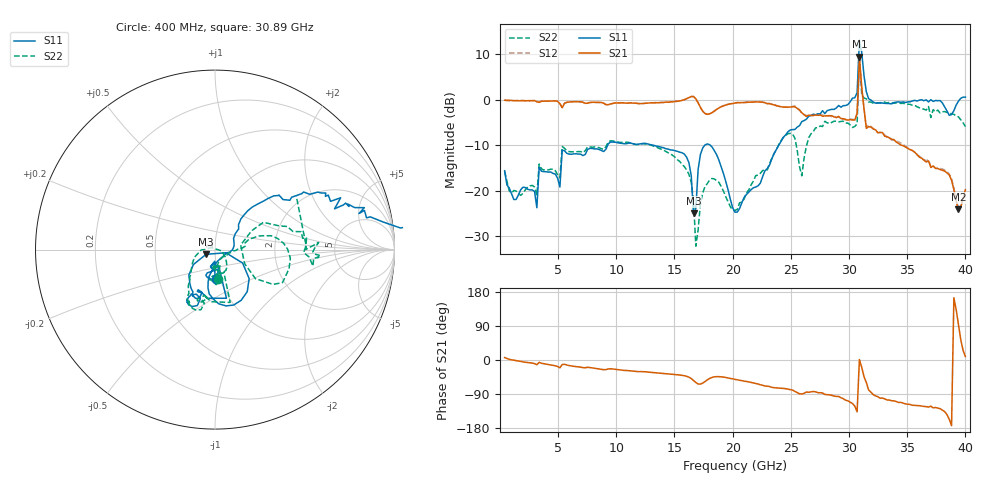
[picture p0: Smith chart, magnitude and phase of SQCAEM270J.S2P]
! Network Analyzer HP8722ES.07.66: Jul 25, 2000 Serial No. US39175408
! 27 Oct 2004  10:19:02
! Frequency  S11  S21  S12  S22
# HZ  S  DB R  50
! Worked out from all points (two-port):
!   201 points, 400 MHz to 40 GHz, reference 50 ohm
!   highest |S21| = 9.46 dB at 30.89 GHz (marker M1); lowest = -24.1 dB at 39.41 GHz (marker M2)
!   |S21| within 3 dB of the highest: 30.84443 GHz to 30.98179 GHz (137.4 MHz wide, 0.444 % of centre)
!   lowest |S11| = -25.0 dB at 16.64 GHz (marker M3), VSWR 1.12, Z = 45.2 - j2.37 ohm
!   |S11| at or under -10 dB: start of sweep to 9.261 GHz; 13.13 GHz to 17.61 GHz (4.482 GHz wide, 29.2 % of centre); 18.06 GHz to 23.97 GHz (5.905 GHz wide, 28.1 % of centre)
!   |S22| runs from -32.3 to 9.5 dB; largest |S21 - S12| = 1.4
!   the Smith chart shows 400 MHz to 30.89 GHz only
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4e8  -15.64 -88.1  -0.12 6.4  -0.05 7.5  -15.78 -84.0
3.172e9  -23.79 -90.8  -0.44 -12.4  -0.43 -12.6  -21.06 -71.2
3.37e9  -14.89 -90.2  -0.57 -6.3  -0.55 -6.5  -14.17 -87.9
7.132e9  -12.30 -112.7  -0.55 -20.1  -0.59 -20.4  -11.65 -103.2
1.3666e10  -10.33 -118.8  -0.67 -34.6  -0.62 -34.7  -10.71 -120.7
1.6042e10  -12.67 -127.3  0.23 -43.1  0.22 -43.1  -15.44 -140.9
1.6636e10  -25.05 -152.2  0.70 -54.3  0.71 -53.8  -22.21 -178.2
1.6834e10  -23.94 -16.3  0.18 -59.3  0.21 -59.9  -32.26 153.6
1.7824e10  -9.74 -71.4  -3.22 -52.4  -3.20 -52.4  -18.46 -57.0
2.02e10  -24.78 -54.3  -0.73 -51.2  -0.74 -51.1  -24.39 -48.7
2.4754e10  -7.05 42.4  -1.65 -76.8  -1.68 -76.6  -7.48 -6.6
2.5942e10  -4.81 32.8  -2.88 -89.7  -2.97 -89.3  -16.75 10.2
2.6932e10  -3.19 27.1  -3.46 -83.1  -3.51 -83.9  -7.00 13.1
3.0694e10  1.55 -6.5  -3.02 -136.8  -3.00 -135.2  -5.32 33.2
3.0892e10  13.05 14.2  9.46 1.1  6.95 -24.9  9.48 -71.6
3.109e10  10.44 4.9  2.85 -19.1  2.54 -19.4  1.31 -33.1
3.1288e10  5.29 -24.6  -2.01 -43.9  -2.00 -44.1  0.37 -18.4
3.1486e10  1.77 -21.0  -6.32 -59.3  -5.94 -61.0  0.20 -12.5
3.3466e10  -0.84 -28.6  -8.42 -105.6  -8.40 -104.8  -0.57 -22.9
3.7822e10  -0.18 -44.5  -15.37 -128.5  -15.14 -128.5  -2.92 -51.2
3.9406e10  -0.31 -14.7  -24.14 92.9  -23.77 97.5  -3.78 -71.5
4e10  0.57 -22.1  -19.83 9.2  -20.18 13.0  -5.93 -77.4
